(* Logix 5000 DataType export R4AO8DIDO_Seneca_OutData; software revision 35.00 *)

TYPE R4AO8DIDO_Seneca_OutData :   // User Define Data Out Type for Seneca R-4AO-8DIDO-E Device
STRUCT
   DOUT1 : BOOL;   // Digital Output1
   DOUT2 : BOOL;   // Digital Output2
   DOUT3 : BOOL;   // Digital Output3
   DOUT4 : BOOL;   // Digital Output4
   DOUT5 : BOOL;   // Digital Output5
   DOUT6 : BOOL;   // Digital Output6
   DOUT7 : BOOL;   // Digital Output7
   DOUT8 : BOOL;   // Digital Output8
   AO1 : REAL;   // Analog Output 1
   AO2 : REAL;   // Analog Output 2
   AO3 : REAL;   // Analog Output 3
   AO4 : REAL;   // Analog Output 4
   CMD : INT;   // Command Register
   CMD_AUX : UDINT;   // Command Auxiliar
END_STRUCT
END_TYPE
